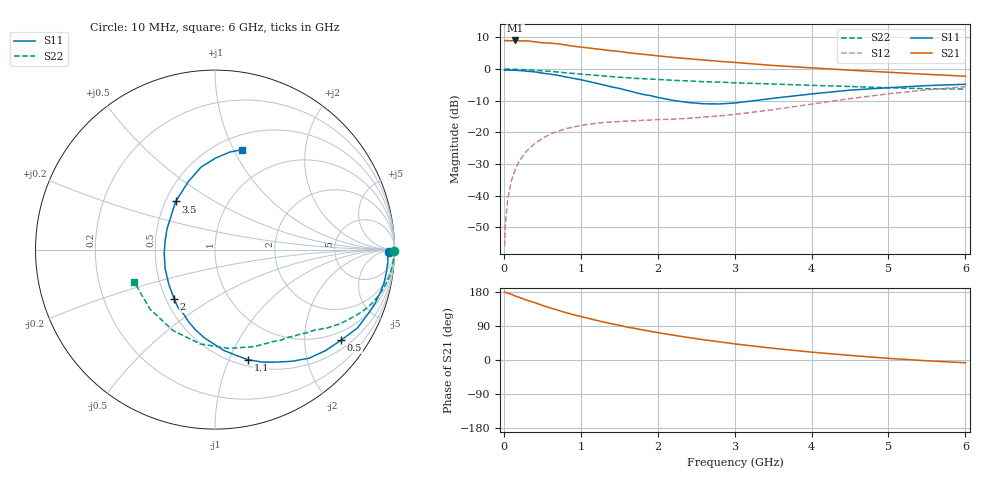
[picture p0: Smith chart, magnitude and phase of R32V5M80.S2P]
! SIEMENS Small Signal Semiconductors
! BFR181
! Si NPN RF Bipolar Junction Transistor in SOT23
! VCE = 2.5 V  IC = 0.8 mA
! Common Emitter S-Parameters:  May  1996
# GHz  S  MA  R  50
!  f  S11  S21  S12  S22
! GHz  MAG  ANG  MAG  ANG  MAG  ANG  MAG  ANG
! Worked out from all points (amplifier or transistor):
!   36 points, 10 MHz to 6 GHz, reference 50 ohm
!   highest |S21| = 9.1 dB at 150 MHz (marker M1)
!   |S21| within 3 dB of that: start of sweep to 1.321 GHz
!   unconditionally stable (mu >= 1): 2.122 GHz to 3.762 GHz
!   at 250 MHz: K = 0.14, MSG = 18.1 dB, |S12| = -27.3 dB
!   at 1.4 GHz: K = 0.71, MSG = 11.2 dB, |S12| = -16.7 dB
!   at 6 GHz: K = 0.89, MSG = 1.7 dB, |S12| = -5.5 dB
!   S11 on the Smith chart (normalised r, x): 10 MHz: 55, -21; 500 MHz: 0.73, -2.94; 1.1 GHz: 0.57, -1.17; 2 GHz: 0.55, -0.35; 3.5 GHz: 0.56, +0.34; 6 GHz: 0.65, +1.08
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0.01  0.9686 -0.7  2.797 179.6  0.0016 97.9  0.9994 -0.4
0.02  0.9614 -1.4  2.827 178.4  0.0035 86.0  0.9992 -0.8
0.05  0.9659 -3.8  2.824 176.5  0.0089 87.4  0.9983 -1.7
0.1  0.9633 -7.3  2.802 173.2  0.0176 86.4  0.9958 -3.4
0.15  0.9601 -11.0  2.839 168.6  0.0264 82.2  0.9919 -5.2
0.3  0.9279 -22.1  2.798 157.7  0.0514 75.8  0.9766 -10.1
0.4  0.906 -28.8  2.705 151.6  0.0666 71.1  0.961 -13.4
0.5  0.865 -35.7  2.605 144.0  0.0805 67.3  0.9429 -16.2
0.6  0.8345 -42.4  2.578 137.7  0.0936 62.8  0.9237 -19.0
0.7  0.8005 -49.1  2.512 131.5  0.1042 59.2  0.9016 -21.6
0.8  0.7566 -55.3  2.414 125.4  0.1139 55.7  0.8774 -24.0
0.9  0.7171 -60.9  2.306 119.7  0.1218 53.0  0.8555 -26.1
1.1  0.6397 -73.4  2.164 109.8  0.1348 48.1  0.8172 -29.9
1.4  0.5246 -90.9  1.95 95.6  0.1464 43.0  0.7642 -34.8
1.6  0.4623 -103.2  1.828 87.0  0.1514 41.2  0.7332 -37.3
2  0.3575 -129.5  1.622 72.3  0.1599 40.4  0.6892 -42.3
2.2  0.3212 -143.4  1.534 65.6  0.1622 41.4  0.6668 -45.1
2.8  0.2821 169.9  1.33 48.1  0.1825 45.7  0.6249 -53.9
3.5  0.3463 129.2  1.144 30.9  0.2292 50.3  0.5829 -68.1
4.5  0.4662 99.6  0.963 12.1  0.3419 47.7  0.532 -98.9
5.5  0.5497 81.4  0.828 -2.1  0.4715 35.1  0.4912 -137.6
6  0.5771 74.7  0.774 -7.3  0.529 27.1  0.4845 -158.0
